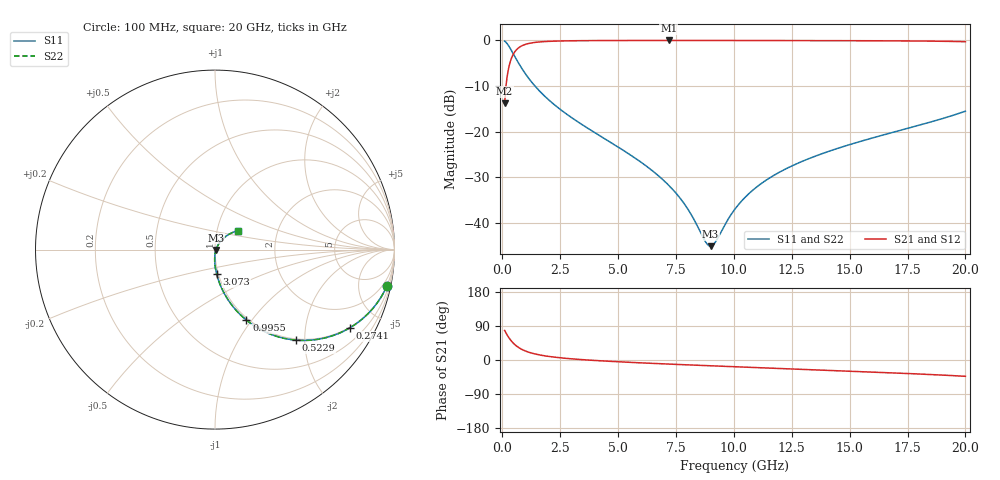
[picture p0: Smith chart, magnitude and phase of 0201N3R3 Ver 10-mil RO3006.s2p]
# GHz S MA R 50
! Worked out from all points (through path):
!   1601 points, 100 MHz to 20 GHz, reference 50 ohm
!   highest |S21| = -0.05 dB at 7.189 GHz (marker M1); lowest = -13.8 dB at 100 MHz (marker M2)
!   group delay of S21, straight-line fit = 8.9 ps
!   lowest |S11| = -45.1 dB at 8.993 GHz (marker M3), VSWR 1.01, Z = 50.5 - j0.163 ohm
!   |S11| at or under -10 dB: 1.408 GHz to end of sweep
!   |S22| runs from -45.1 to -0.2 dB; largest |S21 - S12| = 0
!   S11 on the Smith chart (normalised r, x): 100 MHz: 0.98, -9.49; 274.1 MHz: 0.98, -3.46; 522.9 MHz: 0.98, -1.81; 995.5 MHz: 0.98, -0.94; 3.073 GHz: 0.98, -0.28; 20 GHz: 1.27, +0.28
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0.1  0.979 -11.9  0.2035 78.1  0.2035 78.1  0.979 -11.9
0.274125  0.8683 -30.1  0.4951 59.8  0.4951 59.8  0.8683 -30.1
0.3860625  0.7789 -39.4  0.626 50.5  0.626 50.5  0.7789 -39.4
0.522875  0.6753 -48.3  0.7362 41.6  0.7362 41.6  0.6753 -48.3
0.7343125  0.545 -58.1  0.8369 31.8  0.8369 31.8  0.545 -58.1
0.9955  0.4305 -66.0  0.9008 23.8  0.9008 23.8  0.4305 -66.0
1.716875  0.2608 -77.3  0.963 12.2  0.963 12.2  0.2608 -77.3
3.072563  0.1379 -86.0  0.9872 2.7  0.9872 2.7  0.1379 -86.0
3.420812  0.1205 -87.3  0.9893 1.1  0.9893 1.1  0.1205 -87.3
5.62225  0.05372 -91.9  0.9941 -6.5  0.9941 -6.5  0.05372 -91.9
6.741625  0.03296 -91.3  0.9945 -9.6  0.9945 -9.6  0.03296 -91.3
7.189375  0.02586 -89.8  0.9946 -10.8  0.9946 -10.8  0.02586 -89.8
7.898313  0.01573 -83.3  0.9945 -12.6  0.9945 -12.6  0.01573 -83.3
8.7565  0.006362 -44.9  0.9943 -14.7  0.9943 -14.7  0.006362 -44.9
8.992812  0.005588 -16.7  0.9942 -15.3  0.9942 -15.3  0.005588 -16.7
9.216688  0.006277 9.6  0.9941 -15.8  0.9941 -15.8  0.006277 9.6
10.05  0.01424 47.4  0.9937 -17.8  0.9937 -17.8  0.01424 47.4
10.63456  0.02082 53.5  0.9933 -19.2  0.9933 -19.2  0.02082 53.5
11.36838  0.02916 56.3  0.9928 -20.9  0.9928 -20.9  0.02916 56.3
13.37081  0.05222 56.4  0.991 -25.6  0.991 -25.6  0.05222 56.4
16.69162  0.09559 50.6  0.9853 -33.5  0.9853 -33.5  0.09559 50.6
20  0.1676 39.2  0.9629 -43.0  0.9629 -43.0  0.1676 39.2
